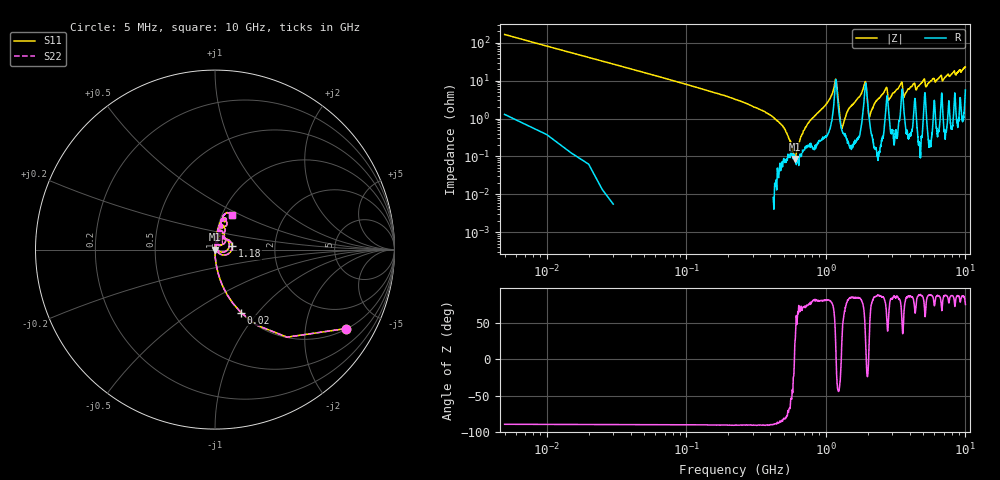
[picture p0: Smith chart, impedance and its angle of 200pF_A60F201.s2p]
! Amotech Co.,Ltd.
! http://www.amotech.co.kr/
! Part Number: A60F201
! These Parameters are Measured in Series Mode Connection
! Operation Temp=25[degC], DC Bias Voltage=0[V]
! Freq. Start=5[MHz] Stop=10[GHz], 2000[Steps]
! Date: Monday, July 20, 2020, 03:47:52
# GHZ S RI R 50.000000
!Freq.(Hz) S11(Real) S11(Imag) S21(Real) S21(Imag) S12(Real) S12(Imag) S22(Real) S22(Imag)
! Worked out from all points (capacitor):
!   2000 points, 5 MHz to 10 GHz, reference 50 ohm
!   read as one part in series: C = 194 pF near 55 MHz
!   lowest |Z| = 85.3 mohm at 600 MHz (marker M1)
!   series resonance near 596 MHz, so ESL is about 370 pH
!   S11 on the Smith chart (normalised r, x): 5 MHz: 1.03, -3.30; 20 MHz: 1.00, -0.82; 1.18 GHz: 1.21, +0.05; 10 GHz: 1.11, +0.44
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0.005  0.7304 -0.4399  0.2696 0.4399  0.2696 0.4399  0.7304 -0.4399
0.02  0.1441 -0.3505  0.8559 0.3505  0.8559 0.3505  0.1441 -0.3505
0.065  0.0151 -0.1232  0.9849 0.1232  0.9849 0.1232  0.0151 -0.1232
0.12  0.00398 -0.0657  0.996 0.0657  0.996 0.0657  0.00398 -0.0657
0.45  0.000565 -0.00848  0.9994 0.00848  0.9994 0.00848  0.000565 -0.00848
0.6  0.000792 0.000314  0.9992 -0.000314  0.9992 -0.000314  0.000792 0.000314
0.76  0.00204 0.00803  0.998 -0.00803  0.998 -0.00803  0.00204 0.00803
1.18  0.0965 0.021  0.9035 -0.021  0.9035 -0.021  0.0965 0.021
1.315  0.0044 0.00378  0.9956 -0.00378  0.9956 -0.00378  0.0044 0.00378
1.675  0.00395 0.0322  0.9961 -0.0322  0.9961 -0.0322  0.00395 0.0322
1.91  0.064 0.0571  0.936 -0.0571  0.936 -0.0571  0.064 0.0571
2.07  0.00686 0.00939  0.9931 -0.00939  0.9931 -0.00939  0.00686 0.00939
2.69  0.02 0.058  0.98 -0.058  0.98 -0.058  0.02 0.058
2.84  0.0125 0.029  0.9875 -0.029  0.9875 -0.029  0.0125 0.029
3.34  0.0128 0.0649  0.9872 -0.0649  0.9872 -0.0649  0.0128 0.0649
3.495  0.0479 0.0731  0.9521 -0.0731  0.9521 -0.0731  0.0479 0.0731
3.635  0.0155 0.0331  0.9845 -0.0331  0.9845 -0.0331  0.0155 0.0331
5.005  0.0216 0.0993  0.9784 -0.0993  0.9784 -0.0993  0.0216 0.0993
5.235  0.0193 0.0653  0.9807 -0.0653  0.9807 -0.0653  0.0193 0.0653
6.67  0.0379 0.128  0.9621 -0.128  0.9621 -0.128  0.0379 0.128
8.335  0.0595 0.1626  0.9405 -0.1626  0.9405 -0.1626  0.0595 0.1626
10  0.0934 0.1902  0.9066 -0.1902  0.9066 -0.1902  0.0934 0.1902
